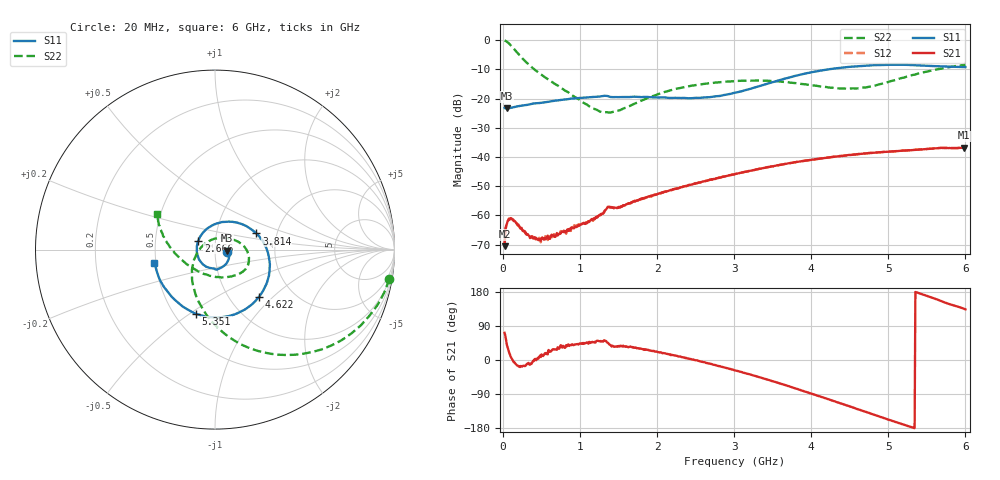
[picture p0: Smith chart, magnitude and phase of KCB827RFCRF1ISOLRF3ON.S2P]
!Agilent Technologies,E5071B,JP1KK00126,A.08.11
!Date: Tue May 06 07:35:28 2014
!Data & Calibration Information:
!Freq	S11:SOLT2(ON)	S21:SOLT2(ON)	S12:SOLT2(ON)	S22:SOLT2(ON)
# Hz S dB R 50
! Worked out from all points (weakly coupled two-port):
!   600 points, 20 MHz to 6 GHz, reference 50 ohm
!   highest |S21| = -36.80 dB at 5.98 GHz (marker M1); lowest = -70.5 dB at 20 MHz (marker M2)
!   lowest |S11| = -23.4 dB at 49.95 MHz (marker M3), VSWR 1.15, Z = 57.2 - j0.651 ohm
!   |S11| at or under -10 dB: start of sweep to 4.222 GHz
!   |S22| runs from -24.8 to -0.1 dB; largest |S21 - S12| = 0.00013
!   S11 on the Smith chart (normalised r, x): 20 MHz: 1.14, -0.03; 2.666 GHz: 0.83, +0.08; 3.814 GHz: 1.56, +0.30; 4.622 GHz: 1.36, -0.82; 5.351 GHz: 0.64, -0.53; 6 GHz: 0.49, -0.08
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2e7  -23.18 -12.6  -70.51 71.6  -70.53 66.0  -0.13 -9.6
4.994992e7  -23.39 -4.8  -62.86 39.6  -62.82 39.0  -0.58 -23.3
7.989983e7  -23.28 -3.5  -61.17 19.1  -61.07 18.4  -1.24 -35.7
1.397997e8  -22.96 -4.0  -61.95 -6.1  -61.74 -3.9  -2.99 -56.0
2.196661e8  -22.51 -6.1  -64.25 -18.6  -64.22 -17.0  -5.39 -75.7
3.194992e8  -22.15 -12.0  -66.41 -10.2  -66.65 -15.2  -8.05 -93.2
5.09182e8  -21.39 -22.0  -67.53 13.1  -68.16 13.2  -12.10 -118.0
1.018331e9  -19.76 -58.7  -63.09 43.0  -63.12 43.6  -21.02 -177.5
1.25793e9  -19.31 -78.6  -59.74 48.9  -59.98 48.8  -24.46 137.9
1.397696e9  -19.49 -92.6  -57.29 38.6  -57.14 39.7  -24.75 106.0
1.507513e9  -19.53 -99.6  -57.31 37.2  -57.21 36.4  -24.11 84.0
2.016661e9  -19.64 -142.7  -52.58 20.7  -52.67 20.5  -18.44 26.7
2.665576e9  -19.55 151.8  -47.99 -8.9  -47.93 -8.8  -14.78 -4.2
3.014992e9  -18.01 109.3  -45.79 -27.5  -45.82 -27.8  -14.04 -18.2
3.444274e9  -14.81 58.5  -43.45 -52.5  -43.42 -52.4  -13.95 -34.1
3.813656e9  -12.13 21.3  -41.68 -76.3  -41.67 -76.3  -14.78 -52.0
4.013322e9  -10.96 3.2  -40.90 -89.7  -40.93 -89.8  -15.49 -65.1
4.622304e9  -8.88 -47.2  -38.97 -131.0  -39.00 -131.3  -16.48 -123.8
5.011653e9  -8.46 -77.9  -38.17 -158.0  -38.15 -158.4  -14.21 -163.0
5.351085e9  -8.57 -106.5  -37.57 179.4  -37.58 179.2  -11.76 174.5
5.980033e9  -9.25 -165.7  -36.80 135.4  -36.79 135.3  -8.47 149.0
6e9  -9.24 -167.7  -36.82 133.8  -36.77 133.8  -8.43 148.4
